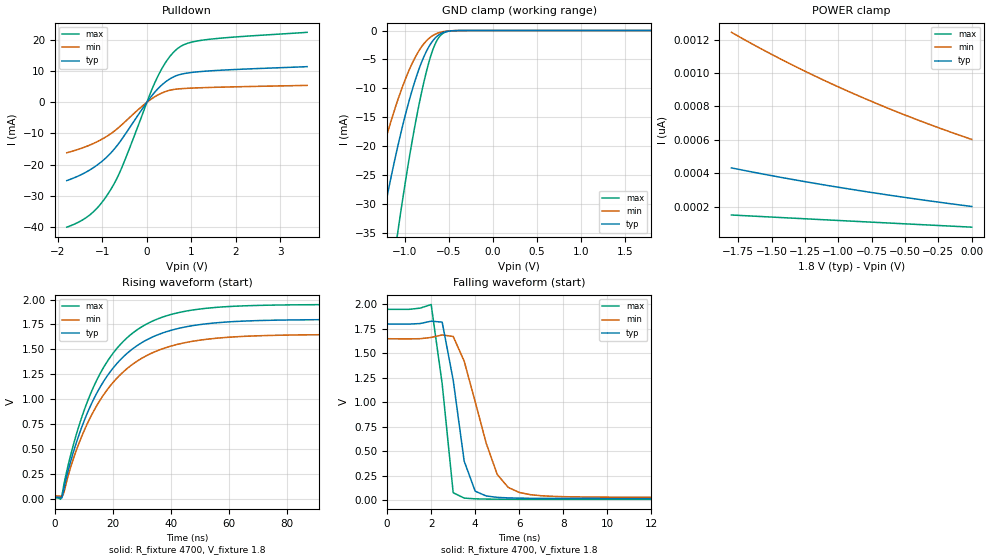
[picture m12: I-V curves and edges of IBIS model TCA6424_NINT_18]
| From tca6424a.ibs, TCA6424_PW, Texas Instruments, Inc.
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[Model]   TCA6424_NINT_18
Model_type  Open_drain
Enable   Active-Low
Vref =   1.8
Rref =   4700
Cref =   50p
Vmeas =   0.9
| variable   typ   min   max
C_comp   2.34pF   1.77pF   2.59pF
| C_pulldown   3.40pF   2.39pF   4.41pF
| C_tri-state   2.34pF   1.77pF   2.59pF
[Temperature Range]   40   100   -40
| Ambient temperature   25   85   -40
[Voltage range]   1.8   1.65   1.95
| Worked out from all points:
|   slope of the pulldown table from 0 to 0.27 V, typ, clamps not added: 57.8 ohm
|   GND clamp passes 1 mA (typ) near -0.63 V on its own axis
|   rising waveform, R_fixture 4700, V_fixture 1.8: 20-80 % time 18.8ns typ, 19.8ns min, 17.9ns max; typ from 0.019 V to 1.8 V
|   falling waveform, R_fixture 4700, V_fixture 1.8: 20-80 % time 722ps typ, 1.24ns min, 586ps max; typ from 1.8 V to 0.019 V
[GND Clamp]
| TCA6424_NINT_18
|   Voltage   I(typ)   I(min)   I(max)
-1.8V     -83.85mA   -57.85mA   -128.1mA
-1.475V   -51.91mA   -34.44mA   -82.81mA
-1.275V   -34.61mA   -22.1mA    -57.29mA
-1.165V   -26.11mA   -16.17mA   -44.36mA
-1.075V   -19.79mA   -11.86mA   -34.51mA
-950mV    -12.15mA   -6.843mA   -22.19mA
-860mV    -7.631mA   -4.054mA   -14.53mA
-770mV    -4.111mA   -2.06mA    -8.117mA
-685mV    -1.851mA   -905.8uA   -3.5mA
-600mV    -617.3uA   -324.3uA   -953.9uA
-475mV    -64.69uA   -46.59uA   -65.3uA
1.8V      200.5pA    643.6pA    70.87pA
[POWER Clamp]
| TCA6424_NINT_18
|   Voltage   I(typ)   I(min)   I(max)
-1.8V     431.5pA    1.243nA    149.6pA
-1.595V   399.5pA    1.152nA    141.1pA
-1.37V    366.3pA    1.058nA    131.9pA
-1.17V    338.4pA    979.8pA    123.7pA
-945mV    308.7pA    897pA      114.6pA
-715mV    280.1pA    817.6pA    105.3pA
-485mV    253pA      743.4pA    96.09pA
-245mV    226.3pA    670.9pA    86.52pA
-16.28fV  200.5pA    601.9pA    76.8pA
[Pulldown]
| TCA6424_NINT_18
|   Voltage   I(typ)   I(min)   I(max)
-1.8V     -25.1mA    -16.18mA   -40.03mA
-1.255V   -21.44mA   -13.54mA   -35.78mA
-1.045V   -19.33mA   -12.1mA    -32.72mA
-825mV    -16.46mA   -10.19mA   -28.27mA
-550mV    -11.56mA   -7.016mA   -20.47mA
60mV      1.174mA    652.4uA    2.253mA
215mV     3.846mA    2.097mA    7.413mA
445mV     6.827mA    3.573mA    13.29mA
680mV     8.622mA    4.255mA    17.11mA
920mV     9.403mA    4.495mA    18.95mA
1.315V    9.977mA    4.717mA    20.05mA
3.6V      11.43mA    5.425mA    22.44mA
[Ramp]
| TCA6424_NINT_18
| variable   typ   min   max
dV/dt_r   1.07/1.88E-08   0.97/1.98E-08   1.17/1.79E-08
dV/dt_f   1.10/6.76E-10   1.00/1.23E-09   1.19/4.03E-10
R_load = 4700
[Rising Waveform]
| TCA6424_NINT_18
R_fixture =   4700
C_fixture =   0
L_fixture =   0
V_fixture =   1.8
V_fixture_min = 1.65
V_fixture_max = 1.95
|   Time   V(typ)   V(min)   V(max)
0s        18.95mV    31.09mV    10.71mV
2.5ns     13.38mV    26.48mV    42.4mV
5.5ns     380.5mV    322.1mV    444.2mV
10ns      775.3mV    677.6mV    880mV
14.5ns    1.063V     938.5mV    1.194V
20ns      1.31V      1.166V     1.459V
32ns      1.601V     1.443V     1.76V
49.5ns    1.747V     1.591V     1.903V
98.5ns    1.799V     1.648V     1.949V
520ns     1.8V       1.65V      1.95V
[Falling Waveform]
| TCA6424_NINT_18
R_fixture =   4700
C_fixture =   0
L_fixture =   0
V_fixture =   1.8
V_fixture_min = 1.65
V_fixture_max = 1.95
|   Time   V(typ)   V(min)   V(max)
0s        1.8V       1.65V      1.95V
2ns       1.829V     1.663V     1.999V
2.5ns     1.819V     1.688V     1.19V
3ns       1.228V     1.673V     78.19mV
3.5ns     399.6mV    1.42V      23.25mV
4.5ns     44.98mV    582.1mV    13.26mV
5ns       30.83mV    264.8mV    12.16mV
6ns       22.75mV    80.9mV     11.26mV
10ns      19.19mV    32.84mV    10.76mV
520ns     18.95mV    31.09mV    10.71mV
